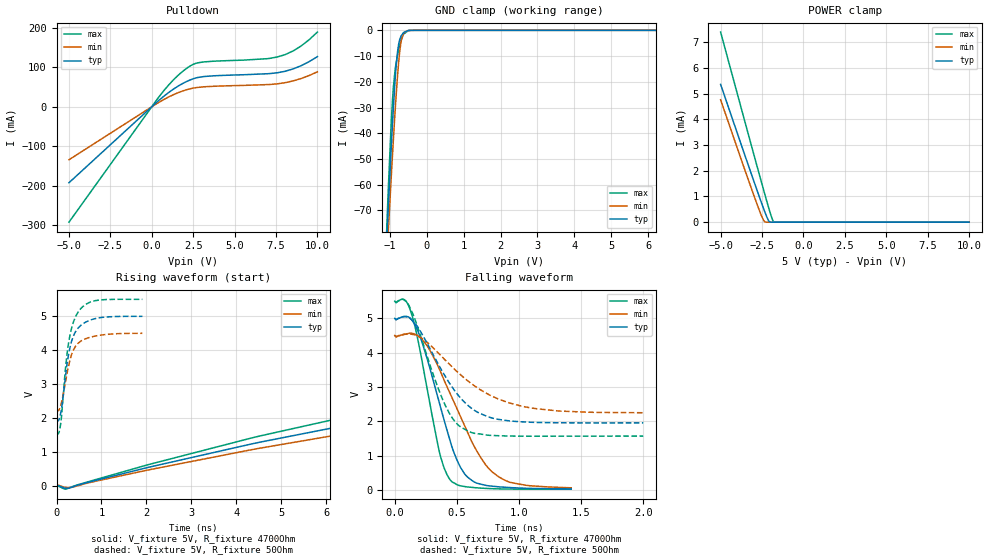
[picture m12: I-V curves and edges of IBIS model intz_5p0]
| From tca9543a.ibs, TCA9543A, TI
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|   intz_5p0 Model
[Model]   intz_5p0
Model_type   Open_drain
Polarity   Non-Inverting
Vmeas = 2.5
Vref = 5
Cref = 100pF
Rref = 4700
|   typ   min   max
|   (nom PVT)   (fast PVT)   (slow PVT)
C_comp   1.561e-12   1.437e-12   1.842e-12
| Where nom  PVT is Nominal Process, 5V, 27C
|   Fast PVT is Strong Process,  5.5V, -40C
|   Slow PVT is Weak Process,   4.5V, 85C
[Voltage Range]   5   4.5   5.5
|Junction Temperature
[Temperature Range]   27   85   -40
[Pullup Reference]   5   4.5   5.5
[Pulldown Reference]   0   0   0
[Power Clamp Reference]   5   4.5   5.5
[GND Clamp Reference]   0   0   0
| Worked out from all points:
|   slope of the pulldown table from 0 to 0.75 V, typ, clamps not added: 27.4 ohm
|   GND clamp passes 1 mA (typ) near -0.63 V on its own axis
|   POWER clamp passes 1 mA (typ) near -2.67 V on its own axis
|   falling waveform, V_fixture 5V, R_fixture 4700Ohm: 20-80 % time 238ps typ, 344ps min, 174ps max; typ from 5 V to 0.027 V
|   rising waveform, V_fixture 5V, R_fixture 4700Ohm: 20-80 % time 17.6ns typ, 18.4ns min, 16.7ns max; typ from 0.027 V to 5 V
|   falling waveform, V_fixture 5V, R_fixture 50Ohm: 20-80 % time 317ps typ, 469ps min, 234ps max; typ from 5 V to 1.95 V
|   rising waveform, V_fixture 5V, R_fixture 50Ohm: 20-80 % time 229ps typ, 245ps min, 218ps max; typ from 1.96 V to 5 V
[Pulldown]
|   Voltage   I(typ)   I(min)   I(max)
-5V       -192.4mA   -134.2mA   -292.3mA
418mV     15.86mA    10.96mA    24.26mA
1.3V      44.48mA    30.44mA    67.78mA
2.046V    62.82mA    42.41mA    95.53mA
2.524V    71.25mA    47.43mA    107.9mA
3.095V    76.27mA    50.36mA    113.4mA
7.006V    83.74mA    56.22mA    121.9mA
7.606V    86.32mA    58.24mA    126.4mA
8.063V    90.07mA    61.18mA    132.3mA
8.536V    95.91mA    65.57mA    141.5mA
9.013V    103.9mA    71.53mA    153.9mA
10V       127mA      88.5mA     189.2mA
[GND Clamp]
|   Voltage   I(typ)   I(min)   I(max)
-5V       -1.565A    -1.407A    -1.822A
-1.115V   -92.54mA   -99.26mA   -89.44mA
-1.07V    -78.39mA   -86.65mA   -72.71mA
-1.04V    -69.17mA   -78.4mA    -61.95mA
-963mV    -46.51mA   -57.88mA   -36.81mA
-908mV    -31.66mA   -43.98mA   -23.22mA
-851mV    -18.37mA   -30.54mA   -14.96mA
-795mV    -8.986mA   -18.81mA   -10.08mA
-690mV    -2.123mA   -4.08mA    -3.731mA
-626mV    -843.5uA   -1.01mA    -1.499mA
-500mV    -84.61uA   -61.47uA   -116uA
10V       0A         0A         0A
[POWER Clamp]
|   Voltage   I(typ)   I(min)   I(max)
-5V       5.358mA    4.761mA    7.393mA
-3.042V   1.685mA    1.129mA    2.747mA
-2.494V   683.1uA    190.9uA    1.46mA
-2.327V   393.1uA    16.9uA     1.076mA
-2.09V    46.6uA     13.29nA    540.8uA
-2.02V    6.958uA    0A         388.8uA
-1.876V   31.71nA    0A         106.1uA
-1.788V   0A         0A         9.811uA
10V       0A         0A         0A
[Ramp]
R_load = 4700
|   typ   min   max
dV/dt_r   2.9839/1.75973e-08   2.67913/1.844e-08   3.28844/1.67625e-08
dV/dt_f   2.9839/2.38277e-10   2.67913/3.46191e-10   3.28844/1.74063e-10
[Falling Waveform]
V_fixture = 5V
V_fixture_min = 4.5V
V_fixture_max = 5.5V
R_fixture = 4700Ohm
|   Time   V(typ)   V(min)   V(max)
0s        5V         4.5V       5.5V
80ps      5.058V     4.538V     5.535V
140ps     4.937V     4.562V     5.072V
220ps     4.3V       4.383V     3.746V
360ps     2.52V      3.513V     1.087V
450ps     1.373V     2.771V     271.6mV
590ps     356.9mV    1.644V     81.02mV
730ps     132.2mV    736.3mV    41.29mV
830ps     88.88mV    393.8mV    27.62mV
1.42ns    26.59mV    57.93mV    18.76mV
[Rising Waveform]
V_fixture = 5V
V_fixture_min = 4.5V
V_fixture_max = 5.5V
R_fixture = 4700Ohm
|   Time   V(typ)   V(min)   V(max)
0s        26.83mV    34.78mV    19.27mV
210ps     -54.82mV   -31.3mV    -79.67mV
4.33ns    1.245V     1.076V     1.421V
6.46ns    1.803V     1.561V     2.052V
11.26ns   2.794V     2.435V     3.165V
18.25ns   3.739V     3.285V     4.206V
27.01ns   4.396V     3.896V     4.912V
36.34ns   4.749V     4.232V     5.271V
47.36ns   4.928V     4.412V     5.444V
100ns     5V         4.5V       5.5V
[Falling Waveform]
V_fixture = 5V
V_fixture_min = 4.5V
V_fixture_max = 5.5V
R_fixture = 50Ohm
|   Time   V(typ)   V(min)   V(max)
0s        5V         4.5V       5.5V
70ps      5.047V     4.529V     5.548V
120ps     5.007V     4.543V     5.333V
230ps     4.471V     4.387V     4.241V
390ps     3.407V     3.841V     2.594V
470ps     2.952V     3.554V     2.058V
540ps     2.635V     3.322V     1.809V
740ps     2.146V     2.809V     1.597V
1.04ns    1.98V      2.425V     1.563V
2ns       1.953V     2.247V     1.566V
[Rising Waveform]
V_fixture = 5V
V_fixture_min = 4.5V
V_fixture_max = 5.5V
R_fixture = 50Ohm
|   Time   V(typ)   V(min)   V(max)
0s        1.955V     2.255V     1.566V
50ps      1.95V      2.239V     1.573V
90ps      2.132V     2.365V     1.82V
210ps     3.347V     3.142V     3.606V
280ps     3.962V     3.608V     4.311V
370ps     4.399V     3.994V     4.809V
480ps     4.655V     4.207V     5.123V
640ps     4.824V     4.338V     5.345V
870ps     4.936V     4.423V     5.464V
1.91ns    5.001V     4.502V     5.5V
